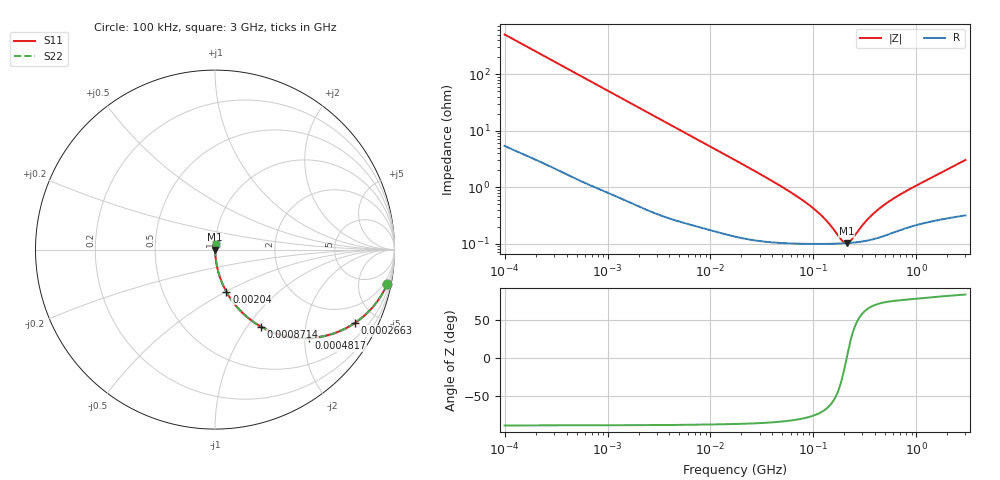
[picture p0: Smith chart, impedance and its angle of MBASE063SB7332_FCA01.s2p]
! MBASE063SB7332_FCA01  S-PARAMETER MODEL  ( Standard Model )
! Model Generated by TAIYO YUDEN Corporation (http://www.ty-top.com)
! Version 1.0
! TAIYO YUDEN Control No. 220601
! Copyright(c) 2020 TAIYO YUDEN CO.,LTD. All Rights Reserved.
! Product Description (link to TY-COMPAS)
! https://ds.yuden.co.jp/TYCOMPAS/or/detail?pn=MBASE063SB7332KFCA01&u=M
! Products Name : Multilayer Ceramic Capacitors
! Characteristics :
!  Capacitance : 3300 [pF] , Rated Voltage : 16 [V] , TCC : X7R
!  Case Size : 0.6 x 0.3 / 0.024 x 0.012 [mm/inch] , Thickness : 0.3 / 0.012 [mm/inch]
!  (Conditions: Temperature = 25 [degC] , DC Bias Voltage = 0 [V])
! External Node Assignments :
!  1  o---| |---o  2
! GND o---------o GND
! Frequency Range : 100kHz  -  3GHz  [ 401 STEP ]
# MHZ S RI R 50
! Freq[MHz].  S11 Real  S11 Imag  S21 Real  S21 Imag  S12 Real  S12 Imag  S22 Real  S22 Imag
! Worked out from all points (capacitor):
!   401 points, 100 kHz to 3 GHz, reference 50 ohm
!   read as one part in series: C = 3.17 nF near 105.3 kHz
!   lowest |Z| = 102 mohm at 211 MHz (marker M1)
!   series resonance near 210.6 MHz, so ESL is about 180 pH
!   S11 on the Smith chart (normalised r, x): 100 kHz: 1, -10; 266.3 kHz: 1.05, -3.79; 481.7 kHz: 1.03, -2.10; 871.4 kHz: 1.02, -1.17; 2.04 MHz: 1.01, -0.50; 3 GHz: 1.01, +0.06
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0.1  0.9597 -0.1913  0.0403 0.1913  0.0403 0.1913  0.9597 -0.1913
0.167439  0.8972 -0.2979  0.1028 0.2979  0.1028 0.2979  0.8972 -0.2979
0.266273  0.7789 -0.4087  0.2211 0.4087  0.2211 0.4087  0.7789 -0.4087
0.481683  0.5248 -0.4926  0.4752 0.4926  0.4752 0.4926  0.5248 -0.4926
0.562235  0.4493 -0.4905  0.5507 0.4905  0.5507 0.4905  0.4493 -0.4905
0.871356  0.2576 -0.4298  0.7424 0.4298  0.7424 0.4298  0.2576 -0.4298
1.316074  0.1351 -0.3336  0.8649 0.3336  0.8649 0.3336  0.1351 -0.3336
2.039661  0.0632 -0.2346  0.9368 0.2346  0.9368 0.2346  0.0632 -0.2346
3.161081  0.0288 -0.1577  0.9712 0.1577  0.9712 0.1577  0.0288 -0.1577
6.674626  0.00806 -0.0768  0.9919 0.0768  0.9919 0.0768  0.00806 -0.0768
17.7727  0.00217 -0.0292  0.9978 0.0292  0.9978 0.0292  0.00217 -0.0292
52.46276  0.00111 -0.00941  0.9989 0.00941  0.9989 0.00941  0.00111 -0.00941
97.38194  0.00101 -0.00426  0.999 0.00426  0.999 0.00426  0.00101 -0.00426
132.6759  0.000996 -0.0024  0.999 0.0024  0.999 0.0024  0.000996 -0.0024
190.323  0.00101 -0.000509  0.999 0.000509  0.999 0.000509  0.00101 -0.000509
210.9903  0.00102 9.12e-06  0.999 -9.12e-06  0.999 -9.12e-06  0.00102 9.12e-06
233.9019  0.00103 0.000528  0.999 -0.000528  0.999 -0.000528  0.00103 0.000528
302.6647  0.0011 0.00186  0.9989 -0.00186  0.9989 -0.00186  0.0011 0.00186
362.5028  0.00118 0.00285  0.9988 -0.00285  0.9988 -0.00285  0.00118 0.00285
547.5153  0.0015 0.00542  0.9985 -0.00542  0.9985 -0.00542  0.0015 0.00542
916.7529  0.00212 0.00952  0.9979 -0.00952  0.9979 -0.00952  0.00212 0.00952
3000  0.00404 0.0298  0.996 -0.0298  0.996 -0.0298  0.00404 0.0298
